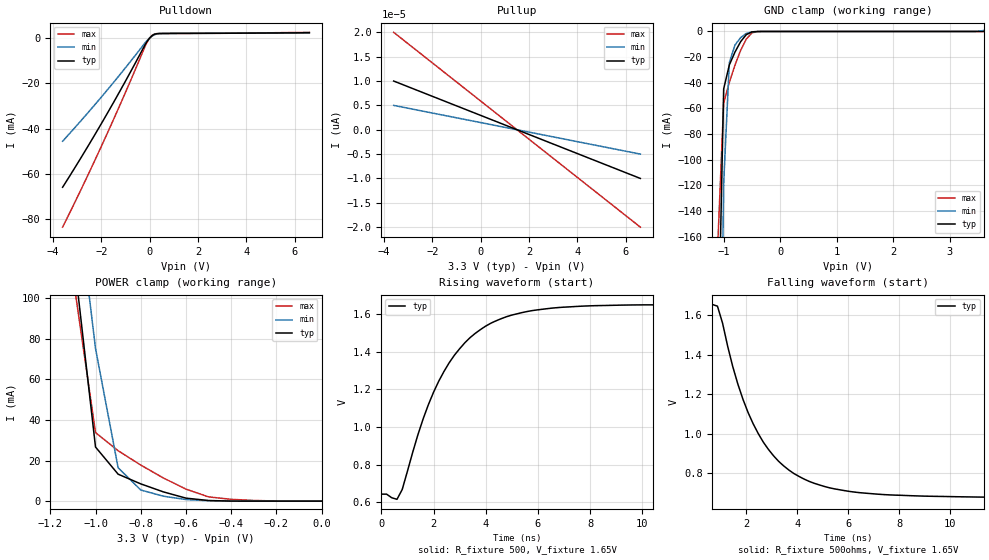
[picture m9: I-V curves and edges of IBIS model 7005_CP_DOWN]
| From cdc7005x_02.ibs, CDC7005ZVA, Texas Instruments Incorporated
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| CHARGE PUMP OUT PULL-DOWN PULSE
[Model]   7005_CP_DOWN
Model_type   3-state
Polarity   Non-Inverting
Enable   Active-High
Vmeas = 1.65V   |Vref for timing measurements.
Cref = 0pF   |load capacitance for timing spec.
Rref = 500ohms   |500 Ohm to VCC/2
Vref = 1.65V   |Timing specification test load voltage; GND
|   typ   min   max
C_comp   2.86pF   2.8pF   2.91pF
[Temperature range]   27   125   -20
[Voltage range]   3.3   3.0   3.6
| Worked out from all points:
|   slope of the pulldown table from 0 to 0.495 V, typ, clamps not added: 252 ohm
|   GND clamp passes 1 mA (typ) near -0.53 V on its own axis
|   POWER clamp passes 1 mA (typ) near -0.56 V on its own axis
|   rising waveform, R_fixture 500, V_fixture 1.65V: 20-80 % time 2.05ns typ, NA min, NA max; typ from 0.644 V to 1.65 V
|   falling waveform, R_fixture 500ohms, V_fixture 1.65V: 20-80 % time 1.99ns typ, NA min, NA max; typ from 1.66 V to 0.668 V
| Notes: (1) Vtable = Vcc - Voutput
|   (2) Pullup data includes the effects of the ESD
|   clamping circuitry
[Pullup]   | Is off for PULL-DOWN Pulse
|   27C:3.3V:nominal   125C:3.0V:weak   -20C:3.6V:strong
|  Voltage   I(typ)   I(min)   I(max)
-3.6V     10pA       5pA        20pA
6.6V      -10pA      -5pA       -20pA
[Pulldown]
|   27C:3.3V:nominal   125C:3.0V:weak   -20C:3.6V:strong
|  Voltage   I(typ)   I(min)   I(max)
-3.6V     -65.9mA    -45.59mA   -83.51mA
-2.7V     -50.41mA   -34.81mA   -63.82mA
-1.9V     -36.01mA   -24.84mA   -45.54mA
-1V       -19.03mA   -13.13mA   -24mA
-200mV    -3.169mA   -2.256mA   -3.915mA
0V        -195.2pA   -646.4pA   -52.06nA
100mV     1.016mA    808.5uA    1.158mA
300mV     1.898mA    1.775mA    1.909mA
500mV     1.962mA    1.993mA    1.951mA
6.6V      2.292mA    2.228mA    2.485mA
[POWER Clamp]
|   27C:3.3V:nominal   125C:3.0V:weak   -20C:3.6V:strong
|  Voltage   I(typ)   I(min)   I(max)
-3.6V     3.248A     2.572A     4.171A
-1.1V     124.2mA    167.9mA    110.9mA
-1V       26.63mA    75.14mA    33.74mA
-900mV    13.27mA    16.44mA    24.83mA
-800mV    8.502mA    5.477mA    17.76mA
-700mV    4.551mA    2.43mA     11.4mA
-600mV    1.477mA    777.7uA    5.912mA
-500mV    299.3uA    201uA      2.081mA
-400mV    26.9uA     28.19uA    894.9uA
-300mV    1.191uA    2.625uA    331.3uA
0V        245.2pA    1.646nA    229.2pA
[GND Clamp]
|   27C:3.3V:nominal   125C:3.0V:weak   -20C:3.6V:strong
|  Voltage   I(typ)   I(min)   I(max)
-3.6V     -12.74A    -10.05A    -16.37A
-1.1V     -253.9mA   -443mA     -161.5mA
-1V       -44.77mA   -118.5mA   -55.73mA
-900mV    -26.11mA   -24.29mA   -39.68mA
-800mV    -16.07mA   -10.54mA   -26.23mA
-700mV    -7.95mA    -4.789mA   -14.73mA
-600mV    -2.456mA   -1.484mA   -5.897mA
-500mV    -327.7uA   -267.2uA   -1.086mA
-400mV    -21.87uA   -33.38uA   -64.02uA
3.3V      245.2pA    2.625uA    -48.88nA
3.6V      1.191uA    777.7uA    229.2pA
[ramp]
| variable   typ   min   max
dV/dt_r   0.5935/2.0610E-09   NA   NA
dV/dt_f   0.5935/1.9971E-09   NA   NA
[Rising Waveform]
R_fixture = 500
V_fixture =  1.65V
|   27C:3.3V:nominal   125C:3.0V:weak  -20C:3.6V:strong
|   Time   V(typ)   V(min)   V(max)
0s        643.9mV    NA         NA
600ps     616.3mV    NA         NA
800ps     668.1mV    NA         NA
1.8ns     1.118V     NA         NA
2.2ns     1.243V     NA         NA
2.8ns     1.381V     NA         NA
3.6ns     1.497V     NA         NA
4.8ns     1.586V     NA         NA
8.2ns     1.644V     NA         NA
19.6ns    1.651V     NA         NA
[Falling Waveform]
R_fixture = 500ohms
V_fixture =  1.65V
V_fixture_min = 1.5V
V_fixture_max = 1.8V   | Plot was truncated to
|   allow faster simulation periodes.
|   27C:3.3V:nominal   125C:3.0V:weak -20C:3.6V:strong
|   Time   V(typ)   V(min)   V(max)
661ps     1.656V     NA         NA
861ps     1.647V     NA         NA
1.661ns   1.253V     NA         NA
2.061ns   1.109V     NA         NA
2.461ns   1.002V     NA         NA
3.261ns   860.7mV    NA         NA
4.461ns   758.8mV    NA         NA
5.861ns   711.6mV    NA         NA
7.661ns   689.9mV    NA         NA
19.66ns   667.6mV    NA         NA
